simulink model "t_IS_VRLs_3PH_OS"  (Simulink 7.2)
settings: Solver=ode3  StartTime=0.0  StopTime=0.02  FixedStep=1e-5  RelTol=1e-3

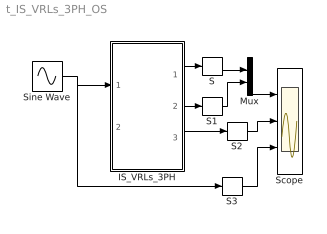
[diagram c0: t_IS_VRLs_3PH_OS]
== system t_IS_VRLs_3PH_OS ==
  IS_VRLs_3PH : Subsystem  mask(IS_VRLs_3PH_OS){R=1, L=1e-3, RLp=1e6}
      mask prompts: R "Res"; L "Inductance"; RLp "Ind. Parallel RLp"
      mask help: Open source IS_VRLs_3PH_OS Input Vector: u[0]= Is, Source Current u[1]= IL, Load Current Output Vector: y[0]=IL123, Inductance current y[1]=VL123, Inductance Voltage y[2]=iR123, Resistance current Parameter Vector: p[0]=R p[1]=L p[2]=IL0 p[3]=RLp
  Mux : Mux  Inputs=2
  S{,1..3} (4 alike) : Selector  InputPortWidth=3  IndexOptions=Index vector (dialog)  Indices=[1 ]  OutputSizes=1
  Scope : Scope  NumInputPorts=3
  Sine Wave : Sin  Amplitude=100  Frequency=1000*pi  Phase="[0  -2*pi/3  -4*pi/3]"  SampleTime=0
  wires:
  Sine Wave/1 -> IS_VRLs_3PH/1(IS123), S3/1
  IS_VRLs_3PH/1(iL123) -> S/1
  Mux/1 -> Scope/1
  IS_VRLs_3PH/2(vL123) -> S1/1
  IS_VRLs_3PH/3(iR123) -> S2/1
  S/1 -> Mux/1
  S1/1 -> Mux/2
  S2/1 -> Scope/2
  S3/1 -> Scope/3

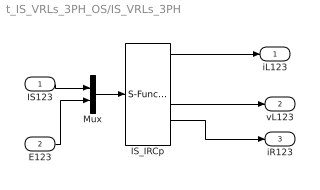
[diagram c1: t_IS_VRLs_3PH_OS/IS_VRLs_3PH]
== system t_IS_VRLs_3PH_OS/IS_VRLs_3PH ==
  IS123 : Inport
  E123 : Inport  Port=2
  IS_IRCp : S-Function  FunctionName=s_IS_VRLs_3PH_OS  Parameters=[R, L, RLp]  EnableBusSupport=off
  Mux : Mux  Inputs=2
  iL123 : Outport
  vL123 : Outport  Port=2
  iR123 : Outport  Port=3
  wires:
  IS_IRCp/1 -> iL123/1
  IS_IRCp/2 -> vL123/1
  Mux/1 -> IS_IRCp/1
  IS123/1 -> Mux/1
  E123/1 -> Mux/2
  IS_IRCp/3 -> iR123/1
